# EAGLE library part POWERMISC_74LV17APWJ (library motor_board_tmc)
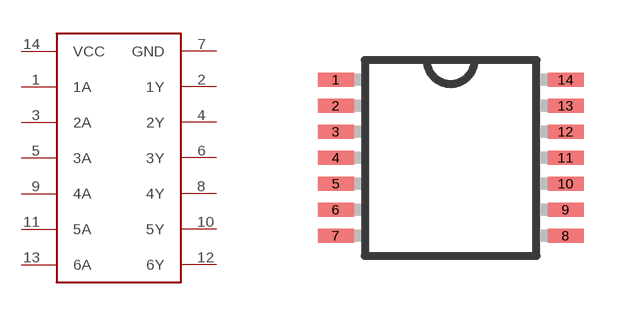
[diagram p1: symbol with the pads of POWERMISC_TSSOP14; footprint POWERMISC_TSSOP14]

Designator prefix U

## POWERMISC_74LV17APWJ  [POWERMISC_TSSOP14]
1  1A
2  1Y
3  2A
4  2Y
5  3A
6  3Y
7  GND
8  4Y
9  4A
10  5Y
11  5A
12  6Y
13  6A
14  VCC

## Footprint POWERMISC_TSSOP14 (pad centres in mm)
14-Lead Thin Shrink Small Outline Package [TSSOP] Source: Analog Devices .. 780914713ADD8704_0.pdf
smd 0.9 x 0.35: 1 -2.875,1.95; 2 -2.875,1.3; 3 -2.875,0.65; 4 -2.875,0; 5 -2.875,-0.65; 6 -2.875,-1.3; 7 -2.875,-1.95; 8 2.875,-1.95; 9 2.875,-1.3; 10 2.875,-0.65; 11 2.875,0; 12 2.875,0.65; 13 2.875,1.3; 14 2.875,1.95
